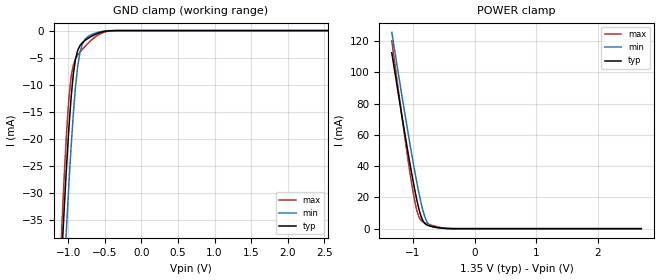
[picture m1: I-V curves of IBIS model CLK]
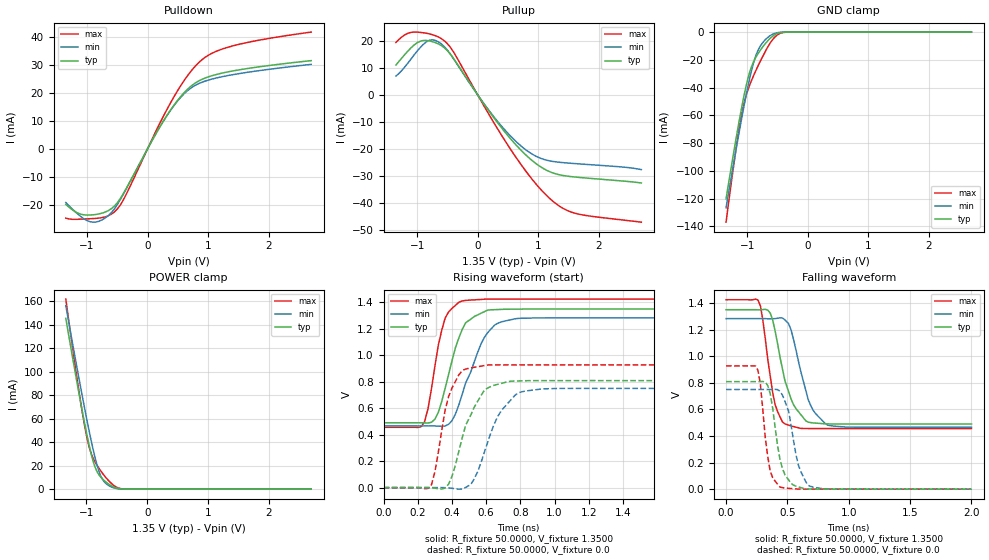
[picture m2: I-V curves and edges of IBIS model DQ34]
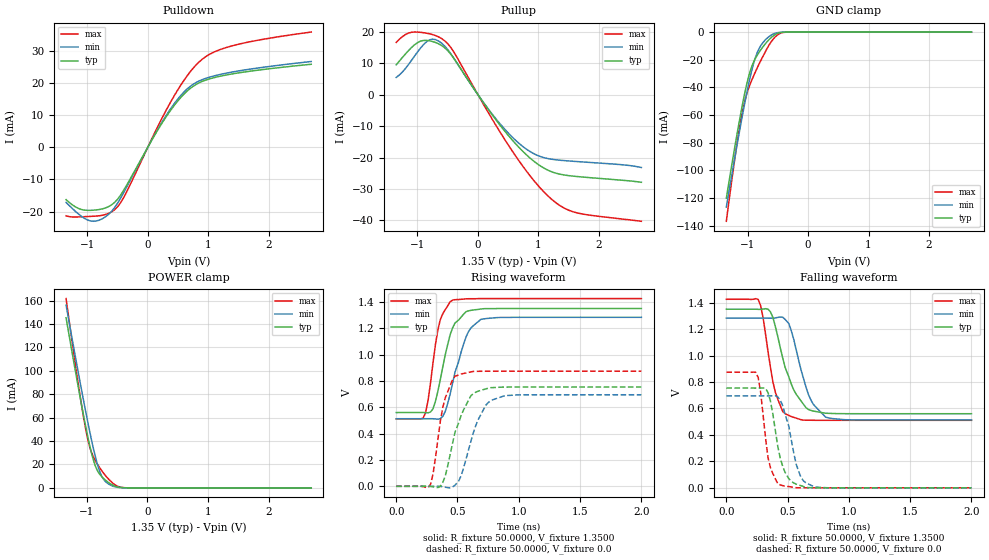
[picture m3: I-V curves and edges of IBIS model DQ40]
|   IBIS file usslh2g16ei.ibs
[IBIS ver] 3.2
[File name] usslh2g16ei.ibs
[File Rev] 1.06
[Date] Dec. 08th, 2020
[Source] File generated by UniIC.
[Notes]  Rev 1.0: 03/21/2019
   - New model generated.
   Rev 1.01: 06/12/2019
   - Adjust DQ34/DQ40 model rising waveform and
   falling waveform.
   Rev 1.02: 10/03/2019
   - 1. Modify CLK and INPUT model GND Clamp and POWER Clamp.
   - 2. Moidfy DQ34 and DQ40 model.
   Rev 1.03: 12/06/2019
   - Modified all ODT model content. Change to use v1.0 value.
   Rev 1.04: 12/06/2019
   - Update RLC information.
   Rev 1.05: 12/23/2019
   - Modified content of all ODT models.
   Rev 1.06: 12/08/2020
   - add -40c data.
   - update 95c data.
[Disclaimer]  THESE IBIS MODELS ARE PROVIDED "AS IS" WITH NO WARRANTY
   AND UniIC IS NOT RESPONSIBLE FOR ANY PROBLEMS THIS MODEL
   MAY CAUSE TO THE CUSTOMERS. THESE MODELS ARE SUBJECT TO CHANGE
   WITHOUT ANY NOTICE.
[Copyright] Copyright 2020. UniIC All rights reserved.
|   Component: SCB13H2G160EF
|   2G DDR3L SDRAM X16
|   VDD/VDDQ : 1.35V
[Component] SCB13H2G160EF
[Manufacturer]  UniIC.
[Package]
|   typ   min   max
R_pkg   0.624   0.464   0.798
L_pkg   1.862nH   1.145nH   3.060nH
C_pkg   0.529pF   0.376pF   0.813pF
[Pin]   signal_name   model_name   R_pin   L_pin   C_pin
A1   VDDQ   POWER
A2   DQU5   DQ   0.782   2.212nH   0.593pF
A3   DQU7   DQ   0.720   1.890nH   0.554pF
A7   DQU4   DQ   0.536   1.899nH   0.568pF
A8   VDDQ   POWER
A9   VSS   GND
B1   VSS   GND
B2   VDD   POWER
B3   VSS   GND
B7   DQSUB   DQ   0.674   1.734nH   0.587pF
B8   DQU6   DQ   0.791   2.263nH   0.576pF
B9   VSS   GND
C1   VDDQ   POWER
C2   DQU3   DQ   0.669   1.891nH   0.538pF
C3   DQU1   DQ   0.577   1.375nH   0.563pF
C7   DQSU   DQ   0.678   1.680nH   0.578pF
C8   DQU2   DQ   0.759   2.136nH   0.557pF
C9   VDDQ   POWER
D1   VSS   GND
D2   VDDQ   POWER
D3   DMU   DQ   0.570   1.24nH   0.562pF
D7   DQU0   DQ   0.511   1.214nH   0.532pF
D8   VSS   GND
D9   VDD   POWER
E1   VSS   GND
E2   VSS   GND
E3   DQL0   DQ   0.527   1.246nH   0.558pF
E7   DML   DQ   0.528   1.181nH   0.559pF
E8   VSS   GND
E9   VDDQ   POWER
F1   VDDQ   POWER
F2   DQL2   DQ   0.649   1.448nH   0.569pF
F3   DQSL   DQ   0.600   1.602nH   0.552pF
F7   DQL1   DQ   0.503   1.145nH   0.544pF
F8   DQL3   DQ   0.610   1.407nH   0.554pF
F9   VSS   GND
G1   VSS   GND
G2   DQL6   DQ   0.589   1.311nH   0.543pF
G3   DQSLB   DQ   0.595   1.638nH   0.544pF
G7   VDD   POWER
G8   VSS   GND
G9   VSS   GND
H1   VREFQ   POWER
H2   VDD   POWER
H3   DQL4   DQ   0.550   1.26nH   0.565pF
H7   DQL7   DQ   0.587   1.352nH   0.567pF
H8   DQL5   DQ   0.731   1.671nH   0.576pF
H9   VDDQ   POWER
J2   VSS   GND
J3   RASB   INPUT   0.464   1.391nH   0.444pF
J7   CK   CLK   0.472   1.167nH   0.376pF
J8   VSS   GND
K1   ODT   INPUT   0.628   2.345nH   0.451pF
K2   VDD   POWER
K3   CASB   INPUT   0.476   1.52nH   0.452pF
K7   CKB   CLK   0.467   1.314nH   0.389pF
K8   VDD   POWER
K9   CKE   INPUT   0.685   2.271nH   0.502pF
L2   CSB   INPUT   0.576   2.026nH   0.444pF
L3   WEB   INPUT   0.495   1.669nH   0.437pF
L7   A10   INPUT   0.491   1.335nH   0.448pF
L8   ZQ   INPUT   0.652   1.676nH   0.497pF
M1   VSS   GND
M2   BA0   INPUT   0.601   2.209nH   0.446pF
M3   BA2   INPUT   0.565   1.827nH   0.450pF
M9   VSS   GND
N1   VDD   POWER
N2   A3   INPUT   0.669   2.297nH   0.501pF
N3   A0   INPUT   0.546   1.663nH   0.460pF
N7   A12   INPUT   0.545   1.919nH   0.480pF
N8   BA1   INPUT   0.671   2.186nH   0.501pF
N9   VDD   POWER
P1   VSS   GND
P2   A5   INPUT   0.701   2.412nH   0.530pF
P3   A2   INPUT   0.614   2.102nH   0.542pF
P7   A1   INPUT   0.582   2.095nH   0.521pF
P8   A4   INPUT   0.686   2.439nH   0.542pF
P9   VSS   GND
R1   VSS   GND
R2   A7   INPUT   0.763   2.744nH   0.587pF
R3   A9   INPUT   0.673   2.375nH   0.534pF
R7   A11   INPUT   0.633   2.347nH   0.507pF
R8   A6   INPUT   0.761   2.758nH   0.599pF
R9   VDD   POWER
T1   VSS   GND
T2   RESETB   INPUT   0.798   2.031nH   0.813pF
T3   A13   INPUT   0.752   2.571nH   0.549pF
T7   A14   INPUT   0.717   2.562nH   0.523pF
T8   A8   INPUT   0.798   3.060nH   0.580pF
T9   VSS   GND
|**********************DIFF PIN*********************************************
[Diff_pin]   inv_pin   vdiff   tdelay_typ   tdelay_min   tdelay_max
   J7   K7   0V   0ns   NA   NA
   F3   G3   0V   0ns   NA   NA
   C7   B7   0V   0ns   NA   NA
|   Model Selector
[Model Selector]  DQ
DQ34   34ohm data I/O without ODT
DQ40   40ohm data I/O without ODT
ODT20   Data input with 20ohm ODT
ODT30   Data input with 30ohm ODT
ODT40   Data input with 40ohm ODT
ODT60   Data input with 60ohm ODT
ODT120   Data input with 120ohm ODT
| Models and submodels in the file (14): CLK (Input), INPUT (Input), DQ34 (I/O), DQ40 (I/O), ODT20 (Input), ODT30 (Input), ODT40 (Input), ODT60 (Input), ODT120 (Input), 20ohm_ODT (Dynamic_clamp), 30ohm_ODT (Dynamic_clamp), 40ohm_ODT (Dynamic_clamp), 60ohm_ODT (Dynamic_clamp), 120ohm_ODT (Dynamic_clamp)
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|   Model CLK
[Model]  CLK
Model_type   Input
Polarity   Non-Inverting
Vinl =   0.5750V
Vinh =   0.7750V
| variable   typ   min   max
C_comp   0.4980pF   0.4480pF   0.5480pF
| variable   typ   min   max
[Temperature Range]   45.000   95.000   -40.0000
| variable   typ   min   max
[Voltage Range]   1.35V   1.283V   1.4250V
| variable   typ   min   max
[POWER Clamp Reference] 1.35V   1.283V   1.4250V
| variable   typ   min   max
[GND Clamp Reference]   0.000V   0.000V   0.000V
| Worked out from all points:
|   GND clamp passes 1 mA (typ) near -0.67 V on its own axis
|   POWER clamp passes 1 mA (typ) near -0.64 V on its own axis
[GND_clamp]
|Voltage   I(typ)   I(min)   I(max)
-1.35V    -119.8mA   -132.6mA   -129.4mA
-1.11V    -47.85mA   -60.25mA   -43.69mA
-1.08V    -39.66mA   -51.82mA   -34.37mA
-1.05V    -31.85mA   -43.65mA   -25.8mA
-1.02V    -24.55mA   -35.8mA    -18.34mA
-960mV    -12.39mA   -21.54mA   -8.568mA
-930mV    -8.108mA   -15.48mA   -6.396mA
-870mV    -3.674mA   -6.627mA   -4.532mA
-810mV    -2.286mA   -2.636mA   -3.515mA
-720mV    -1.363mA   -1.035mA   -2.211mA
-390mV    -14.42uA   -7.911uA   -27.31uA
2.7V      0A         0A         0A
[POWER_clamp]
|Voltage   I(typ)   I(min)   I(max)
-1.34V    112.5mA    125.5mA    120.1mA
-1.2V     77.82mA    90.79mA    78.58mA
-1.1V     53.88mA    66.67mA    50.17mA
-1.02V    35.69mA    48.08mA    29.23mA
-960mV    23.14mA    34.83mA    15.98mA
-900mV    12.44mA    22.6mA     7.477mA
-840mV    5.342mA    12.19mA    4.459mA
-780mV    2.549mA    5.064mA    3.31mA
-720mV    1.647mA    1.95mA     2.478mA
-600mV    737.4uA    566.8uA    1.142mA
-360mV    19.27uA    12.95uA    28.6uA
2.7V      0A         0A         0A
|   Model DQ34
[Model]  DQ34
Model_type I/O
Polarity   Non-Inverting
Enable   Active-High
Vinl =   0.5750V
Vinh =   0.7750V
Vmeas =  0.6750V
Cref =   0.0F
Rref =   25.0000
Vref =   0.6750V
| variable   typ   min   max
C_comp   1.0500pF   1.0000pF   1.1000pF
| variable   typ   min   max
[Temperature Range]   45.000   95.000   -40.0000
| variable   typ   min   max
[Voltage Range]   1.35V   1.283V   1.4250V
| variable   typ   min   max
[Pullup Reference]   1.35V   1.283V   1.4250V
| variable   typ   min   max
[Pulldown Reference]   0.000V   0.000V   0.000V
| variable   typ   min   max
[POWER Clamp Reference] 1.35V   1.283V   1.4250V
| variable   typ   min   max
[GND Clamp Reference]   0.000V   0.000V   0.000V
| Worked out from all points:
|   slope of the pulldown table from 0 to 0.203 V, typ, clamps not added: 25.8 ohm
|   slope of the pullup table from 0 to 0.203 V, typ, clamps not added: 31.3 ohm
|   GND clamp passes 1 mA (typ) near -0.50 V on its own axis
|   POWER clamp passes 1 mA (typ) near -0.51 V on its own axis
|   rising waveform, R_fixture 50.0000, V_fixture 1.3500: 20-80 % time 112ps typ, 142ps min, 82.2ps max; typ from 0.49 V to 1.35 V
|   rising waveform, R_fixture 50.0000, V_fixture 0.0: 20-80 % time 130ps typ, 142ps min, 87.7ps max; typ from 0 V to 0.809 V
|   falling waveform, R_fixture 50.0000, V_fixture 1.3500: 20-80 % time 135ps typ, 138ps min, 91.5ps max; typ from 1.35 V to 0.49 V
|   falling waveform, R_fixture 50.0000, V_fixture 0.0: 20-80 % time 84.9ps typ, 97.5ps min, 65.9ps max; typ from 0.809 V to 0 V
[Pulldown]
|Voltage   I(typ)   I(min)   I(max)
-1.35V    -19.97mA   -19.29mA   -24.89mA
-1.15V    -23.09mA   -23.47mA   -25.29mA
-900mV    -23.69mA   -26.34mA   -25.04mA
-700mV    -22.71mA   -24.85mA   -24.42mA
-500mV    -19.4mA    -20.05mA   -21.62mA
-350mV    -14.14mA   -14.28mA   -16.22mA
100mV     3.983mA    3.979mA    4.628mA
350mV     12.96mA    12.88mA    15.33mA
650mV     21.14mA    20.67mA    25.93mA
900mV     24.9mA     23.86mA    31.96mA
1.45V     28.05mA    26.72mA    37.13mA
2.7V      31.59mA    30.25mA    41.82mA
[Pullup]
|Voltage   I(typ)   I(min)   I(max)
-1.35V    11.07mA    6.98mA     19.41mA
-1.15V    16.28mA    11.86mA    22.82mA
-1V       19.27mA    16.18mA    23.22mA
-850mV    20.14mA    19.59mA    22.82mA
-700mV    19.35mA    20.18mA    21.92mA
-400mV    13.51mA    13.42mA    15.9mA
150mV     -4.843mA   -4.665mA   -5.851mA
550mV     -16.41mA   -15.39mA   -20.35mA
900mV     -24.27mA   -21.87mA   -31.22mA
1.2V      -28.46mA   -24.4mA    -38.48mA
1.6V      -30.3mA    -25.34mA   -43.66mA
2.7V      -32.52mA   -27.58mA   -47mA
[GND_clamp]
|Voltage   I(typ)   I(min)   I(max)
-1.35V    -120.2mA   -126.6mA   -136.9mA
-1.23V    -88.34mA   -95.9mA    -97.82mA
-1.14V    -65.66mA   -73.61mA   -71.4mA
-1.08V    -51.6mA    -59.33mA   -56.75mA
-1.02V    -39.02mA   -45.77mA   -45.84mA
-960mV    -28.85mA   -33.36mA   -38.11mA
-900mV    -21.72mA   -22.78mA   -31.76mA
-810mV    -14.7mA    -12.03mA   -23.22mA
-660mV    -6.182mA   -3.801mA   -10.58mA
-510mV    -1.116mA   -502.7uA   -2.242mA
-300mV    -9.735uA   -5.245uA   -17.77uA
2.7V      0A         0A         0A
[POWER_clamp]
|Voltage   I(typ)   I(min)   I(max)
-1.34V    145.4mA    156.2mA    161.8mA
-1.2V     103.8mA    115.9mA    110.3mA
-1.1V     75.06mA    87.82mA    75.66mA
-1.02V    53.32mA    66.13mA    51.11mA
-960mV    38.36mA    50.57mA    36.78mA
-920mV    29.52mA    40.72mA    30.13mA
-860mV    19.05mA    27.19mA    23.4mA
-780mV    11.23mA    13.2mA     16.7mA
-700mV    6.951mA    5.865mA    11.08mA
-560mV    2.052mA    1.298mA    3.566mA
-340mV    28uA       19.06uA    41.51uA
2.7V      0A         0A         0A
[Ramp]
| variable   typ   min   max
dV/dt_r  0.4853/0.1200n   0.4499/0.1421n   0.5564/88.0013p
dV/dt_f  0.5160/0.1249n   0.4903/0.1383n   0.5816/91.2670p
R_load = 50.0000
[Rising Waveform]
R_fixture= 50.0000
V_fixture= 1.3500
V_fixture_min= 1.2830
V_fixture_max= 1.4250
L_fixture= 0.0H
C_fixture= 0.0F
|time   V(typ)   V(min)   V(max)
0s        490mV      465.8mV    455.7mV
240ps     489.3mV    465.8mV    499.7mV
260ps     488.1mV    465.8mV    598.9mV
300ps     517.4mV    465.9mV    918.4mV
360ps     751.1mV    466.1mV    1.281V
400ps     958.8mV    505.9mV    1.355V
460ps     1.196V     706.9mV    1.411V
590ps     1.33V      1.136V     1.424V
690ps     1.347V     1.253V     1.425V
2ns       1.35V      1.283V     1.425V
[Rising Waveform]
R_fixture= 50.0000
V_fixture= 0.0
V_fixture_min= 0.0
V_fixture_max= 0.0
L_fixture= 0.0H
C_fixture= 0.0F
|time   V(typ)   V(min)   V(max)
0s        0V         0V         0V
280ps     -938.2uV   -50.3uV    22.71mV
380ps     26.61mV    -2.235mV   687.6mV
440ps     273.8mV    -11.77mV   852.1mV
480ps     471.5mV    1.462mV    896.2mV
530ps     607.6mV    65.88mV    909.3mV
590ps     737mV      269.6mV    922.4mV
670ps     781.4mV    542.8mV    927.2mV
790ps     806.3mV    717.3mV    927.4mV
2ns       808.8mV    749.8mV    927.4mV
[Falling Waveform]
R_fixture= 50.0000
V_fixture= 1.3500
V_fixture_min= 1.2830
V_fixture_max= 1.4250
L_fixture= 0.0H
C_fixture= 0.0F
|time   V(typ)   V(min)   V(max)
0s        1.35V      1.283V     1.425V
260ps     1.349V     1.283V     1.423V
300ps     1.351V     1.283V     1.269V
360ps     1.325V     1.282V     851.7mV
400ps     1.189V     1.283V     636mV
480ps     815.1mV    1.274V     491.2mV
530ps     677.3mV    1.198V     475.6mV
670ps     503.9mV    672.9mV    456mV
830ps     490.9mV    481mV      455.7mV
2ns       490mV      465.8mV    455.7mV
[Falling Waveform]
R_fixture= 50.0000
V_fixture= 0.0
V_fixture_min= 0.0
V_fixture_max= 0.0
L_fixture= 0.0H
C_fixture= 0.0F
|time   V(typ)   V(min)   V(max)
0s        808.8mV    749.8mV    927.4mV
260ps     808.5mV    749.8mV    893.8mV
280ps     808.7mV    749.9mV    787.7mV
320ps     805.7mV    749.8mV    383.6mV
360ps     718.4mV    749.6mV    134.6mV
440ps     222mV      736.8mV    15.51mV
510ps     69.56mV    586.8mV    6.017mV
590ps     16.7mV     179.9mV    365.2uV
670ps     1.797mV    27.86mV    -71.92uV
2ns       1.662uV    -1.338uV   1.894uV
|   Model DQ40
[Model]  DQ40
Model_type I/O
Polarity   Non-Inverting
Enable   Active-High
Vinl =   0.5750V
Vinh =   0.7750V
Vmeas =  0.6750V
Cref =   0.0F
Rref =   25.0000
Vref =   0.6750V
| variable   typ   min   max
C_comp   1.0500pF   1.0000pF   1.1000pF
| variable   typ   min   max
[Temperature Range]   45.000   95.000   -40.0000
| variable   typ   min   max
[Voltage Range]   1.35V   1.283V   1.4250V
| variable   typ   min   max
[Pullup Reference]   1.35V   1.283V   1.4250V
| variable   typ   min   max
[Pulldown Reference]   0.000V   0.000V   0.000V
| variable   typ   min   max
[POWER Clamp Reference] 1.35V   1.283V   1.4250V
| variable   typ   min   max
[GND Clamp Reference]   0.000V   0.000V   0.000V
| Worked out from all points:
|   slope of the pulldown table from 0 to 0.203 V, typ, clamps not added: 31 ohm
|   slope of the pullup table from 0 to 0.203 V, typ, clamps not added: 36.5 ohm
|   GND clamp passes 1 mA (typ) near -0.50 V on its own axis
|   POWER clamp passes 1 mA (typ) near -0.51 V on its own axis
|   rising waveform, R_fixture 50.0000, V_fixture 1.3500: 20-80 % time 117ps typ, 137ps min, 87.5ps max; typ from 0.56 V to 1.35 V
|   rising waveform, R_fixture 50.0000, V_fixture 0.0: 20-80 % time 143ps typ, 148ps min, 98.6ps max; typ from 0 V to 0.754 V
|   falling waveform, R_fixture 50.0000, V_fixture 1.3500: 20-80 % time 156ps typ, 141ps min, 104ps max; typ from 1.35 V to 0.56 V
|   falling waveform, R_fixture 50.0000, V_fixture 0.0: 20-80 % time 94.4ps typ, 106ps min, 71.5ps max; typ from 0.754 V to 0 V
[Pulldown]
|Voltage   I(typ)   I(min)   I(max)
-1.35V    -16.31mA   -17.17mA   -21.34mA
-1.15V    -19.01mA   -20.69mA   -21.68mA
-950mV    -19.64mA   -22.91mA   -21.52mA
-650mV    -18.49mA   -20.9mA    -20.6mA
-500mV    -16.2mA    -17.43mA   -18.53mA
-400mV    -13.43mA   -14.16mA   -15.71mA
100mV     3.324mA    3.459mA    3.967mA
400mV     12.09mA    12.6mA     14.82mA
650mV     17.49mA    18.14mA    22.22mA
900mV     20.49mA    21.04mA    27.39mA
1.45V     22.99mA    23.58mA    31.82mA
2.7V      25.82mA    26.68mA    35.84mA
[Pullup]
|Voltage   I(typ)   I(min)   I(max)
-1.35V    9.49mA     5.47mA     16.63mA
-1.15V    13.95mA    9.5mA      19.57mA
-1V       16.52mA    13.51mA    19.91mA
-850mV    17.26mA    16.81mA    19.56mA
-700mV    16.59mA    17.5mA     18.8mA
-400mV    11.58mA    11.64mA    13.63mA
150mV     -4.151mA   -4.025mA   -5.015mA
550mV     -14.06mA   -13.18mA   -17.44mA
900mV     -20.81mA   -18.54mA   -26.76mA
1.2V      -24.4mA    -20.49mA   -32.99mA
1.65V     -26.07mA   -21.3mA    -37.67mA
2.7V      -27.88mA   -23.18mA   -40.28mA
[GND_clamp]
|Voltage   I(typ)   I(min)   I(max)
-1.35V    -120.2mA   -126.6mA   -136.9mA
-1.23V    -88.34mA   -95.9mA    -97.82mA
-1.14V    -65.66mA   -73.61mA   -71.4mA
-1.08V    -51.6mA    -59.33mA   -56.75mA
-1.02V    -39.02mA   -45.77mA   -45.84mA
-960mV    -28.85mA   -33.36mA   -38.11mA
-900mV    -21.72mA   -22.78mA   -31.76mA
-810mV    -14.7mA    -12.03mA   -23.22mA
-660mV    -6.182mA   -3.801mA   -10.58mA
-510mV    -1.116mA   -502.7uA   -2.242mA
-300mV    -9.735uA   -5.245uA   -17.77uA
2.7V      0A         0A         0A
[POWER_clamp]
|Voltage   I(typ)   I(min)   I(max)
-1.34V    145.4mA    156.2mA    161.8mA
-1.2V     103.8mA    115.9mA    110.3mA
-1.1V     75.06mA    87.82mA    75.66mA
-1.02V    53.32mA    66.13mA    51.11mA
-960mV    38.36mA    50.57mA    36.78mA
-920mV    29.52mA    40.72mA    30.13mA
-860mV    19.05mA    27.19mA    23.4mA
-780mV    11.23mA    13.2mA     16.7mA
-700mV    6.951mA    5.865mA    11.08mA
-560mV    2.052mA    1.298mA    3.566mA
-340mV    28uA       19.06uA    41.51uA
2.7V      0A         0A         0A
[Ramp]
| variable   typ   min   max
dV/dt_r  0.4523/0.1331n   0.4170/0.1476n   0.5243/98.6582p
dV/dt_f  0.4740/0.1462n   0.4620/0.1406n   0.5489/0.1040n
R_load = 50.0000
[Rising Waveform]
R_fixture= 50.0000
V_fixture= 1.3500
V_fixture_min= 1.2830
V_fixture_max= 1.4250
L_fixture= 0.0H
C_fixture= 0.0F
|time   V(typ)   V(min)   V(max)
0s        560mV      513mV      512.4mV
220ps     560.2mV    513mV      518.5mV
260ps     557.7mV    513mV      652.2mV
300ps     588.3mV    513mV      936.2mV
360ps     811.2mV    513.9mV    1.266V
400ps     998.2mV    568.3mV    1.341V
460ps     1.203V     782.9mV    1.414V
570ps     1.326V     1.135V     1.423V
690ps     1.346V     1.267V     1.425V
2ns       1.35V      1.283V     1.425V
[Rising Waveform]
R_fixture= 50.0000
V_fixture= 0.0
V_fixture_min= 0.0
V_fixture_max= 0.0
L_fixture= 0.0H
C_fixture= 0.0F
|time   V(typ)   V(min)   V(max)
0s        0V         0V         0V
280ps     -1.179mV   -56.53uV   14.26mV
300ps     -4.246mV   187.6uV    92.07mV
380ps     29.65mV    -3.414mV   597.9mV
480ps     412mV      8.256mV    835.8mV
530ps     539mV      81.09mV    852.7mV
610ps     688.6mV    344.4mV    868.7mV
730ps     739.3mV    614.3mV    873.8mV
790ps     749.5mV    657.8mV    873.8mV
2ns       753.8mV    695mV      873.8mV
[Falling Waveform]
R_fixture= 50.0000
V_fixture= 1.3500
V_fixture_min= 1.2830
V_fixture_max= 1.4250
L_fixture= 0.0H
C_fixture= 0.0F
|time   V(typ)   V(min)   V(max)
0s        1.35V      1.283V     1.425V
260ps     1.349V     1.283V     1.423V
300ps     1.351V     1.283V     1.285V
360ps     1.33V      1.282V     910.8mV
400ps     1.219V     1.284V     722.5mV
480ps     909.4mV    1.273V     559.9mV
530ps     784.3mV    1.187V     538.6mV
670ps     592mV      705mV      511mV
810ps     563.8mV    534.8mV    510.2mV
2ns       560mV      513mV      510.2mV
[Falling Waveform]
R_fixture= 50.0000
V_fixture= 0.0
V_fixture_min= 0.0
V_fixture_max= 0.0
L_fixture= 0.0H
C_fixture= 0.0F
|time   V(typ)   V(min)   V(max)
0s        753.8mV    695mV      873.8mV
260ps     753.4mV    695mV      833.6mV
340ps     720.5mV    694.7mV    229mV
380ps     555.1mV    696.2mV    106.9mV
420ps     311.7mV    686.9mV    30.95mV
460ps     162.1mV    620.7mV    16.28mV
510ps     68.5mV     464.9mV    9.458mV
570ps     27.95mV    178.1mV    1.063mV
650ps     3.55mV     36.84mV    -39.59uV
2ns       5.419uV    1.261uV    1.29uV
